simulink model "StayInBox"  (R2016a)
settings: Solver=FixedStepAuto  StartTime=0.0  StopTime=inf  RelTol=1e-3
libraries: miniQ x2

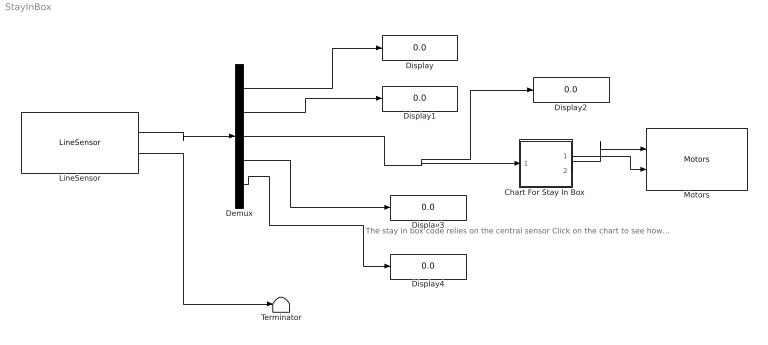
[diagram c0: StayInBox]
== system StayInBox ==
  note: The stay in box code relies on the central sensor Click on the chart to see how the raw values influece the robot's movement
  "Chart For Stay In Box " : Stateflow chart  TreatAsAtomicUnit=on
  Demux : Demux  Outputs=5
  Display{,1..4} (5 alike) : Display
  LineSensor : miniQ/LineSensor  sampleTime_dd=0.01  maxRawSensors=[800,900,900,900,800]  minRawSensors=[200,280,300,300,220]  debug_dd=off
  Motors : miniQ/Motors  flipLeft=off  flipRight=off
  Terminator : Terminator
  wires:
  LineSensor/2 -> Terminator/1
  Demux/1 -> Display/1
  LineSensor/1 -> Demux/1
  Demux/4 -> Display3/1
  Demux/2 -> Display1/1
  Demux/5 -> Display4/1
  Demux/3 -> Display2/1, "Chart For Stay In Box "/1(value)
  "Chart For Stay In Box "/1(r) -> Motors/2
  "Chart For Stay In Box "/2(l) -> Motors/1

== stateflow chart StayInBox/Chart For Stay In Box
 ==
  state Left
    entry: l=-150
    r=150
  state Forward
    entry: l=255
    r=255
  state The entry point is the robot moving forward. The [group]
    threshold value I am using is <300 and this means that the
    robot has hit a black line. It then goes backward for a half second
    then goes left for a half second before moving forward again.
  state Backward
    entry: l=-150
    r=-150
  (default) -> Forward
  Left -> Forward : after(.5,sec)
  Backward -> Left : after(.5,sec)
  Forward -> Backward : [value<900]
  data: value input; r output; l output
